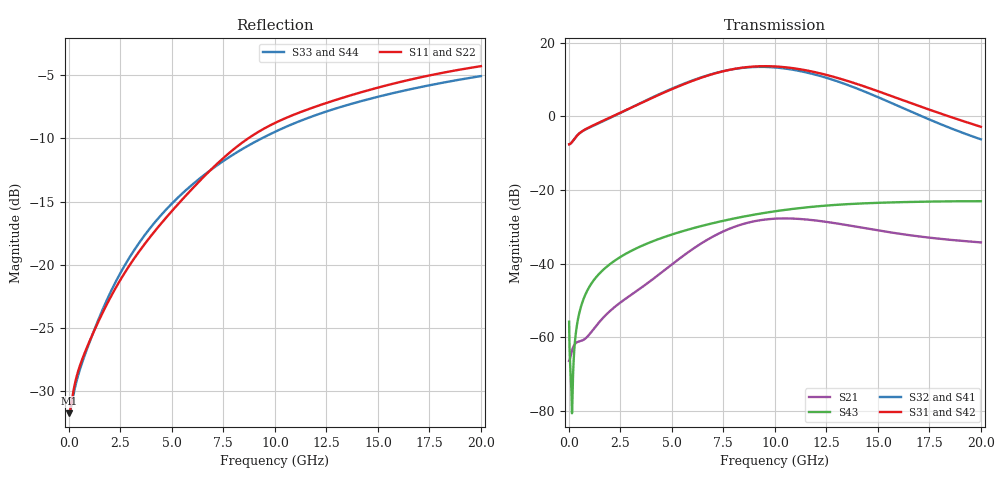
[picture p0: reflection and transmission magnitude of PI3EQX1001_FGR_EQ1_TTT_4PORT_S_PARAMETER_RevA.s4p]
! NPort=4 DATA=2000 NOISE=0 GROUPDELAY=0 COMPLEX_DATAFORMAT=POLAR
! NumOfBlock=1 NumOfParam=0
! .MODEL Smodel S TSTONEFILE=PI3EQX1001_FGR_EQ1_TTT_4PORT_S_PARAMETER_RevA.s4p TYPE=S
!  -- The above .MODEL line can be used for the S element in the netlist.
! The s parameter is extracted from the linear redriver, it is not bi-directional; only s(4,1)s(4,2) and s(3,1)s(3,2)
! should be the insertion loss
!Port definition:
!Port1 = input+
!Port2 = input¨C
!Port3 = output+
!Port4 = output-
# Hz S MA R  50
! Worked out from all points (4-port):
!   2000 points, 10 MHz to 20 GHz, reference 50 ohm
!   strongest paths, dB at 10 MHz, 5.01 GHz, 10.01 GHz, 15.01 GHz, 20 GHz:
!     S31: -7.6, 7.4, 13.5, 6.8, -2.8
!     S42: -7.6, 7.4, 13.5, 6.8, -2.9
!     S32: -7.6, 7.5, 13.3, 5.2, -6.3
!     S41: -7.6, 7.5, 13.2, 5.1, -6.3
!     S43: -55.8, -32.1, -25.8, -23.5, -23.1
!     S21: -66.4, -40.2, -27.8, -31.0, -34.2
!   lowest |S11| = -31.7 dB at 10 MHz (marker M1), VSWR 1.05, Z = 47.5 - j0.063 ohm
!   |S11| at or under -10 dB: start of sweep to 8.703 GHz
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1e7  0.0259 -178.5  0.0004911 2.7  3.669e-05 -0.2  4.787e-05 -0.1
     0.0004778 2.9  0.02597 -178.7  4.577e-05 -0.2  5.994e-05 -0.1
     0.4171 0.3  0.417 -179.7  0.02616 178.4  0.001615 -59.2
     0.4168 -179.7  0.4169 0.3  0.001626 -59.0  0.02612 178.4
6.23e9  0.2098 -104.5  0.01668 99.7  2.299e-05 -30.8  3.285e-05 -29.2
        0.01733 98.0  0.2082 -104.4  3.009e-05 -26.5  4.183e-05 -24.5
        3.198 -48.5  3.239 134.9  0.2156 -111.1  0.0313 61.2
        3.225 134.8  3.193 -48.5  0.0313 61.1  0.2156 -111.1
8.42e9  0.3046 -107.4  0.0332 63.7  2.029e-05 -28.3  3.155e-05 -31.0
        0.03426 62.4  0.3027 -107.5  2.945e-05 -25.7  3.922e-05 -24.8
        4.579 -109.3  4.543 74.4  0.2871 -113.6  0.04325 48.5
        4.517 74.5  4.573 -109.2  0.04315 48.3  0.2869 -113.5
1.051e10  0.3801 -113.5  0.03985 24.6  2.186e-05 -23.3  3.317e-05 -39.4
          0.04106 23.5  0.3773 -113.6  3.15e-05 -33.2  4.013e-05 -24.7
          4.634 -173.1  4.446 11.1  0.3506 -116.9  0.0539 34.6
          4.416 11.2  4.63 -173.0  0.05368 34.5  0.3504 -116.9
1.311e10  0.453 -119.2  0.03367 -10.3  2.828e-05 -37.5  3.088e-05 -61.7
          0.03472 -11.2  0.4492 -119.2  2.914e-05 -53.8  4.529e-05 -35.1
          3.277 114.4  2.936 -60.2  0.4189 -121.4  0.06331 16.5
          2.914 -59.9  3.272 114.5  0.06313 16.6  0.4189 -121.4
1.566e10  0.5183 -123.7  0.02553 -27.2  2.801e-05 -69.1  2.285e-05 -90.8
          0.02641 -28.2  0.514 -123.8  2.07e-05 -79.7  4.245e-05 -56.9
          1.883 57.3  1.516 -114.1  0.476 -125.3  0.06783 0.5
          1.503 -113.6  1.88 57.4  0.06776 0.6  0.4756 -125.3
2e10  0.6102 -131.1  0.01876 -37.1  1.43e-05 -149.8  1.206e-05 151.7
      0.0194 -38.8  0.6048 -131.2  8.114e-06 137.0  1.709e-05 -96.2
      0.7205 -12.1  0.4869 -166.6  0.5574 -131.1  0.07038 -23.6
      0.484 -165.7  0.7184 -11.9  0.07035 -23.6  0.5574 -131.1
